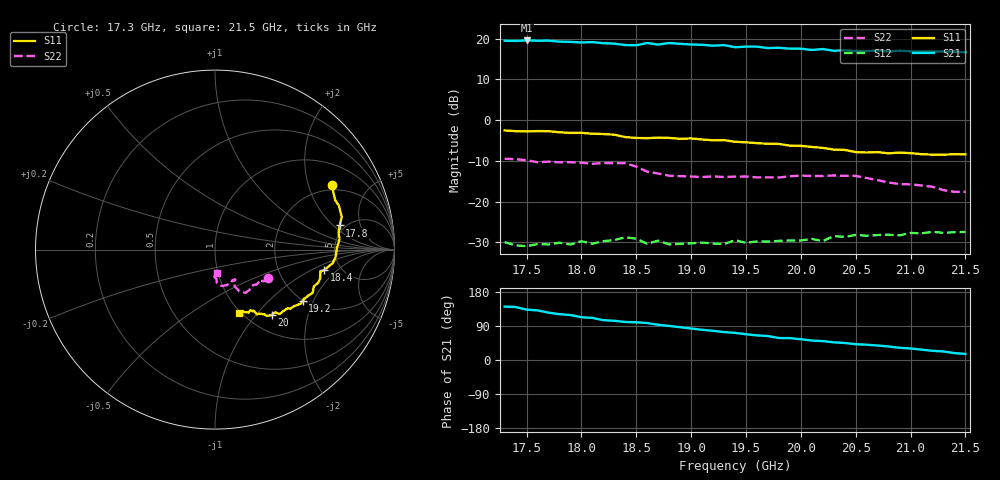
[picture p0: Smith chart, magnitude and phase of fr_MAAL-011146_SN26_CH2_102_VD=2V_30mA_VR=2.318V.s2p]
!Typical measured data - probed
!Date: Friday, August 19, 2022 11:49:57
!Correction: S11(Full 2 Port(1,2))
!S21(Full 2 Port(1,2))
!S12(Full 2 Port(1,2))
!S22(Full 2 Port(1,2))
!S2P File: Measurements: S11, S21, S12, S22:
# Hz S  dB  R 50
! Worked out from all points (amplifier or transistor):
!   43 points, 17.3 GHz to 21.5 GHz, reference 50 ohm
!   highest |S21| = 19.5 dB at 17.5 GHz (marker M1)
!   |S21| within 3 dB of that: start of sweep to end of sweep
!   unconditionally stable (mu >= 1): 17.47647 GHz to 17.5131 GHz; 17.78 GHz to end of sweep
!   at 18 GHz: K = 1.02, MAG = 23.6 dB, |S12| = -29.7 dB
!   at 19.4 GHz: K = 1.47, MAG = 19.6 dB, |S12| = -29.5 dB
!   at 21.5 GHz: K = 1.62, MAG = 17.4 dB, |S12| = -27.5 dB
!   S11 on the Smith chart (normalised r, x): 17.3 GHz: 1.78, +2.88; 17.8 GHz: 4.48, +2.42; 18.4 GHz: 3.68, -1.37; 19.2 GHz: 1.99, -1.66; 20 GHz: 1.28, -1.21; 21.5 GHz: 0.98, -0.81
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1.73e10  -2.55 28.9  19.47 140.9  -29.96 -34.5  -9.50 -27.8
1.74e10  -2.73 25.3  19.40 139.8  -30.75 -39.3  -9.61 -31.7
1.75e10  -2.80 22.2  19.52 132.9  -30.95 -33.9  -9.86 -33.2
1.76e10  -2.71 19.6  19.45 131.0  -30.43 -40.6  -10.36 -34.8
1.78e10  -3.00 11.0  19.24 120.9  -30.10 -36.0  -10.37 -35.5
1.8e10  -3.14 4.9  19.03 112.9  -29.72 -39.0  -10.49 -40.4
1.81e10  -3.36 0.8  19.11 111.1  -30.35 -36.8  -10.74 -43.1
1.82e10  -3.43 -3.4  18.84 105.2  -29.72 -35.1  -10.55 -45.0
1.84e10  -4.19 -10.7  18.39 100.4  -28.77 -39.9  -10.61 -54.8
1.85e10  -4.40 -11.5  18.33 99.5  -29.10 -46.5  -11.42 -59.7
1.86e10  -4.45 -11.5  18.90 97.6  -30.36 -47.2  -12.67 -61.9
1.87e10  -4.33 -15.5  18.51 92.9  -29.60 -46.9  -13.13 -60.1
1.88e10  -4.39 -17.8  18.89 90.0  -30.52 -45.2  -13.67 -57.8
1.92e10  -4.97 -30.2  18.24 77.0  -30.30 -47.0  -13.83 -56.6
1.93e10  -4.93 -31.9  18.38 73.6  -30.44 -43.9  -13.98 -56.8
1.94e10  -5.33 -35.7  17.86 71.6  -29.47 -48.2  -13.89 -58.8
1.98e10  -5.86 -44.9  17.73 58.1  -29.64 -44.5  -14.11 -61.1
2e10  -6.33 -49.1  17.51 54.8  -29.55 -47.2  -13.64 -64.6
2.01e10  -6.60 -52.2  17.18 51.4  -29.16 -49.9  -13.73 -67.6
2.08e10  -8.17 -60.0  16.77 35.7  -28.14 -59.0  -15.34 -86.8
2.09e10  -7.99 -61.9  17.02 32.1  -28.31 -59.3  -15.69 -87.3
2.15e10  -8.43 -69.1  16.60 16.1  -27.46 -67.0  -17.61 -85.4
